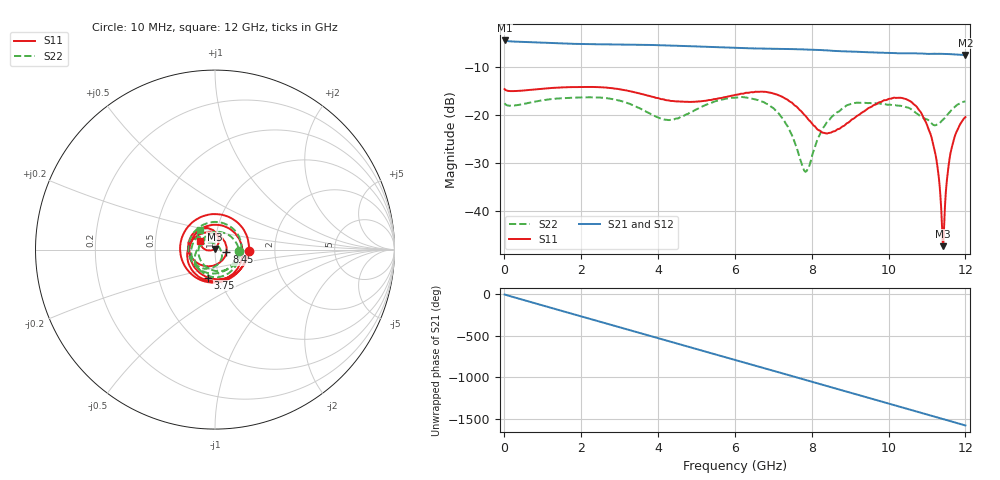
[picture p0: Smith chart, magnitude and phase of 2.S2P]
!Agilent Technologies,E5071C,MY46316741,A.11.02
!Date: Fri Apr 15 15:49:36 2022
!Data & Calibration Information:
!Freq	S11:SOLT2(ON)	S21:SOLT2(ON)	S12:SOLT2(ON)	S22:SOLT2(ON)
!PortZ  Port1:50+j0  Port2:50+j0
!Above PortZ is port z conversion or system Z0 setting when saving the data.
!When reading, reference impedance value at option line is always used.
# Hz S dB R 50
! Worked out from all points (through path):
!   1200 points, 10 MHz to 12 GHz, reference 50 ohm
!   highest |S21| = -4.36 dB at 10 MHz (marker M1); lowest = -7.4 dB at 12 GHz (marker M2)
!   group delay of S21, straight-line fit = 366 ps
!   lowest |S11| = -47.3 dB at 11.42 GHz (marker M3), VSWR 1.01, Z = 49.7 + j0.338 ohm
!   |S11| at or under -10 dB: start of sweep to end of sweep
!   |S22| runs from -31.8 to -16.2 dB; largest |S21 - S12| = 0.0035
!   S11 on the Smith chart (normalised r, x): 10 MHz: 1.46, -0.03; 3.75 GHz: 0.88, -0.28; 8.45 GHz: 1.14, -0.03; 12 GHz: 0.84, +0.08
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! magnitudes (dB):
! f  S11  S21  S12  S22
! 10 MHz  -14.5  -4.4  -4.4  -17.5
! 2.01 GHz  -14.1  -5.1  -5.1  -16.3
! 3.75 GHz  -15.9  -5.3  -5.3  -19.4
! 4.01 GHz  -16.4  -5.3  -5.3  -20.5
! 6.01 GHz  -15.7  -5.9  -5.9  -16.3
! 7.09 GHz  -15.6  -6.1  -6.1  -19.2
! 7.44 GHz  -17.2  -6.2  -6.2  -23.4
! 7.82 GHz  -20.0  -6.2  -6.2  -31.7
! 8.01 GHz  -21.8  -6.3  -6.3  -28.5
! 8.45 GHz  -23.7  -6.5  -6.5  -21.0
! 9.06 GHz  -20.8  -6.7  -6.7  -17.5
! 10.01 GHz  -16.5  -7.0  -7.0  -17.8
! 10.56 GHz  -17.0  -7.1  -7.1  -18.6
! 10.98 GHz  -21.5  -7.2  -7.1  -20.8
! 11.23 GHz  -28.5  -7.2  -7.1  -22.0
! 11.31 GHz  -33.1  -7.1  -7.1  -21.7
! 11.38 GHz  -41.0  -7.2  -7.2  -21.2
! 11.42 GHz  -47.3  -7.2  -7.2  -20.9
! 11.46 GHz  -40.2  -7.2  -7.2  -20.6
! 11.55 GHz  -31.3  -7.2  -7.2  -19.7
! 11.64 GHz  -26.9  -7.2  -7.2  -18.8
! 12 GHz  -20.4  -7.4  -7.4  -17.1
